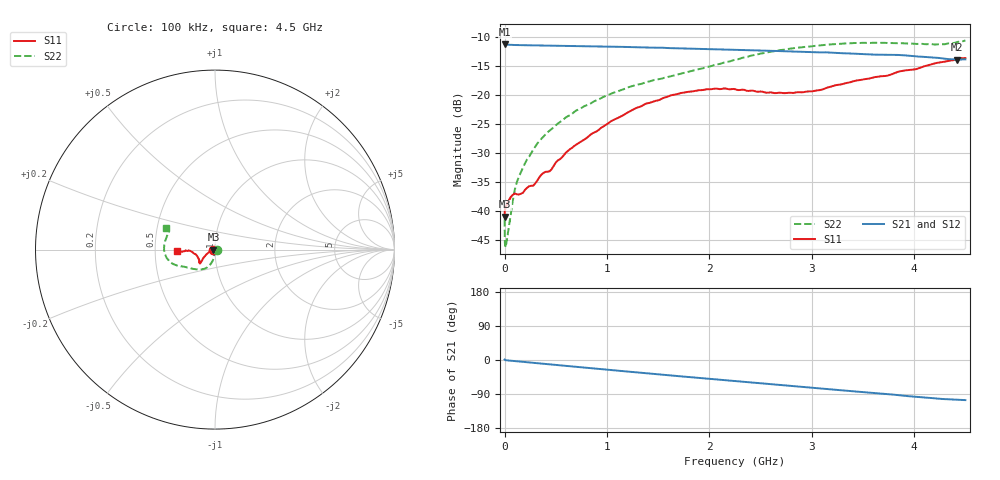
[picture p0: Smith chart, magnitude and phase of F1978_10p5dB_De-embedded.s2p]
! Integrated Device Technology
! Corporate Headquarters
! 6024 Silver Creek Valley Road
! San Jose, CA 95138  USA
! Phone:  1-408-284-8200
! Toll Free:  1-800-223-1366
! Webpage:  http://www.idt.com/
! Timing and RF Division
! 515 Groton Road, Suite 102
! Westford, MA 01886-6024
! Device:  F1978
! Description: 6-bit, 75 ohm, 0.5 dB Digital Step Attenuator
! Frequency:  5.0 MHz -  3.00 GHz
! Package:  4x4 mm QFN Plastic Package: 20 pin
! Ports:  2 RF, 11 DC
!  Pin  1  = D5 (16 dB)
!  Pin  2  = RF1  =  Port 1
!  Pin  3  = Serial Data In (DATA)
!  Pin  4  = Serial Clock (CLK)
!  Pin  5  = Serial Latch Enable (LE)
!  Pin  6  = VDD
!  Pin  7  = NC
!  Pin  8  = NC
!  Pin  9  = NC
!  Pin 10  = GND
!  Pin 11  = GND
!  Pin 12  = NC
!  Pin 13  = VMODE
!  Pin 14  = RF2  =  Port 2
!  Pin 15  = D4 (8 dB)
!  Pin 16  = D3 (4 dB)
!  Pin 17  = D2 (2 dB)
!  Pin 18  = NC
!  Pin 19  = D1 (1 dB)
!  Pin 20  = D0 (0.5 dB)
! State:  21
! Atten State:  10.5 dB
! Voltage:  +3.30 Volts
! Current:  0.562 mA
! Data:  The device was measured on a F1975 evaluation board which has
!  individual transmission lines to the RF pins.  Data was collected
!  using a calibrated network analyzer.  The evaluation board was
!  de-embedded using Automatic Fixture Removal (AFR).
!  The reference plane is the edge of the package pin.
! Misc:
!  Action Tracker AT0416
! Date Measured:  2018-02-08
! Date:  2018-03-26  MJV
! Note:
!  Integrated Device Technology supplies this data as a sample of measured
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# GHz S dB R 75
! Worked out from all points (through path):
!   291 points, 100 kHz to 4.5 GHz, reference 75 ohm
!   highest |S21| = -11.18 dB at 100 kHz (marker M1); lowest = -13.8 dB at 4.42 GHz (marker M2)
!   group delay of S21, straight-line fit = 66.7 ps
!   lowest |S11| = -41.0 dB at 100 kHz (marker M3), VSWR 1.02, Z = 73.7 - j0.00622 ohm
!   |S11| at or under -10 dB: start of sweep to end of sweep
!   |S22| runs from -46.1 to -10.5 dB; largest |S21 - S12| = 0.00018
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0.0001  -41.03 -179.7  -11.18 1.2  -11.18 1.2  -41.50 -2.0
0.0004  -40.67 -177.6  -11.20 1.1  -11.20 1.1  -42.85 -8.7
0.001  -40.18 -176.7  -11.21 1.0  -11.22 1.0  -44.18 -12.4
0.003  -39.77 -176.7  -11.23 0.7  -11.23 0.7  -45.67 -16.9
0.011  -39.35 -175.1  -11.26 -0.5  -11.25 -0.5  -46.13 -43.9
0.08  -37.25 -168.4  -11.31 -2.4  -11.30 -2.4  -38.27 -96.0
0.12  -37.15 -164.2  -11.32 -3.4  -11.32 -3.4  -35.02 -94.8
0.2  -36.36 -166.5  -11.35 -5.5  -11.35 -5.5  -31.76 -95.1
0.32  -34.75 -167.2  -11.39 -8.5  -11.39 -8.5  -28.34 -97.5
0.38  -33.44 -163.2  -11.40 -10.0  -11.40 -10.0  -27.17 -97.5
0.44  -33.17 -162.1  -11.42 -11.5  -11.41 -11.5  -26.12 -97.5
0.52  -31.28 -162.3  -11.44 -13.5  -11.44 -13.5  -24.90 -100.4
0.76  -27.88 -154.8  -11.51 -19.5  -11.50 -19.5  -22.10 -105.5
1.04  -24.50 -149.3  -11.59 -26.5  -11.59 -26.5  -19.75 -112.2
1.52  -20.75 -140.0  -11.78 -38.2  -11.77 -38.2  -17.19 -126.9
1.88  -19.17 -137.2  -11.98 -46.8  -11.98 -46.8  -15.55 -140.5
2.26  -19.01 -139.5  -12.15 -55.7  -12.14 -55.7  -13.83 -152.2
2.64  -19.64 -149.9  -12.34 -64.7  -12.34 -64.7  -12.38 -159.8
3.02  -19.27 -164.9  -12.56 -73.4  -12.55 -73.4  -11.49 -167.5
3.76  -16.51 -177.3  -12.99 -90.3  -12.99 -90.3  -10.97 173.4
4.42  -13.70 -176.0  -13.84 -104.7  -13.84 -104.7  -10.79 157.0
4.5  -13.57 -177.9  -13.79 -105.9  -13.79 -105.9  -10.53 155.6
